FUNCTION F_GetROI : HRESULT
VAR_INPUT
	sFileName 			: 	REFERENCE TO STRING;
	stRoi				:	REFERENCE TO TcVnRectangle_UDINT;
	fThreshold			:	REFERENCE TO LREAL;
	bInvertImage		: 	REFERENCE TO BOOL;
	sPattern			:	REFERENCE TO STRING;
END_VAR
VAR
END_VAR

IF sFileName = 'OCR_01.png' THEN
	stRoi.nX := 86;
	stRoi.nY := 34;
	stRoi.nWidth := 263;
	stRoi.nHeight := 102;
	fThreshold := 150;
	bInvertImage := TRUE;
	sPattern := 'dd#dd#dd';
ELSIF sFileName = 'OCR_02.png' THEN
	stRoi.nX := 69;
	stRoi.nY := 40;
	stRoi.nWidth := 237;
	stRoi.nHeight := 80;
	fThreshold := 150;
	bInvertImage := TRUE;
	sPattern := 'dd#dd#dddd';
ELSIF sFileName = 'OCR_03.png' THEN
	stRoi.nX := 30;
	stRoi.nY := 40;
	stRoi.nWidth := 460;
	stRoi.nHeight := 110;
	fThreshold := 120;
	bInvertImage := TRUE;
	sPattern := 'udddudd###d';
ELSIF sFileName = 'OCR_04.png' THEN
	stRoi.nX := 131;
	stRoi.nY := 25;
	stRoi.nWidth := 243;
	stRoi.nHeight := 83;
	fThreshold := 75;
	bInvertImage := TRUE;
	sPattern := 'dd#dd#dddd';
ELSIF sFileName = 'OCR_05.png' THEN
	stRoi.nX := 129;
	stRoi.nY := 78;
	stRoi.nWidth := 257;
	stRoi.nHeight := 115;
	fThreshold := 150;
	bInvertImage := TRUE;
	sPattern := 'dd#dd#dd';
ELSIF sFileName = 'OCR_06.png' THEN
	stRoi.nX := 71;
	stRoi.nY := 50;
	stRoi.nWidth := 293;
	stRoi.nHeight := 101;
	fThreshold := 75;
	bInvertImage := TRUE;
	sPattern := 'dd#dd#dddd';
ELSIF sFileName = 'OCR_07.png' THEN
	stRoi.nX := 50;
	stRoi.nY := 120;
	stRoi.nWidth := 470;
	stRoi.nHeight := 110;
	fThreshold := 140;
	bInvertImage := FALSE;
	sPattern := 'udddudd###';
ELSIF sFileName = 'OCR_08.png' THEN
	stRoi.nX := 100;
	stRoi.nY := 83;
	stRoi.nWidth := 276;
	stRoi.nHeight := 108;
	fThreshold := 165;
	bInvertImage := TRUE;
	sPattern := 'dd#dd#dd';
ELSIF sFileName = 'OCR_09.png' THEN
	stRoi.nX := 90;
	stRoi.nY := 103;
	stRoi.nWidth := 284;
	stRoi.nHeight := 82; 
	fThreshold := 178;
	bInvertImage := TRUE;
	sPattern := 'dd#dd#dddd';
ELSIF sFileName = 'OCR_10.png' THEN
	stRoi.nX := 207;
	stRoi.nY := 4;
	stRoi.nWidth := 283;
	stRoi.nHeight := 104;
	fThreshold := 130;
	bInvertImage := TRUE;
	sPattern := 'dd#dd#dddd';
ELSIF sFileName = 'OCR_11.png' THEN
	stRoi.nX := 175;
	stRoi.nY := 245;
	stRoi.nWidth := 660;
	stRoi.nHeight := 115;
	fThreshold := 160;
	bInvertImage := TRUE;
	sPattern := 'uu#dddddddd';	
ELSIF sFileName = 'OCR_12.png' THEN 
	stRoi.nX := 74;
	stRoi.nY := 198;
	stRoi.nWidth := 248;
	stRoi.nHeight := 95;
	fThreshold := 130;
	bInvertImage := FALSE;
	sPattern := 'dd#dddd';
ELSIF sFileName = 'OCR_13.png' THEN
	stRoi.nX := 404;
	stRoi.nY := 2;
	stRoi.nWidth := 392;
	stRoi.nHeight := 159;
	fThreshold := 130;
	bInvertImage := FALSE;
	sPattern := 'dd#dd#dd';
ELSIF sFileName = 'OCR_14.png' THEN
	stRoi.nX := 260;
	stRoi.nY := 105;
	stRoi.nWidth := 340;
	stRoi.nHeight := 102;
	fThreshold := 160;
	bInvertImage := FALSE;
	sPattern := 'dd#dd#dddd';
ELSIF sFileName = 'OCR_15.png' THEN
	stRoi.nX := 250;
	stRoi.nY := 5;
	stRoi.nWidth := 560;
	stRoi.nHeight := 125;
	fThreshold := 160;
	bInvertImage := TRUE;
	sPattern := 'uddddd#dd#dd';
ELSIF sFileName = 'OCR_16.png' THEN
	stRoi.nX := 200;
	stRoi.nY := 0;
	stRoi.nWidth := 285;
	stRoi.nHeight := 70;
	fThreshold := 130;
	bInvertImage := FALSE;
	sPattern := 'dd#dd#dddd';
ELSIF sFileName = 'OCR_17.png' THEN
	stRoi.nX := 247;
	stRoi.nY := 83;
	stRoi.nWidth := 213;
	stRoi.nHeight := 94;
	fThreshold := 155;
	bInvertImage := FALSE;
	sPattern := 'dd#dddd';
ELSIF sFileName = 'OCR_18.png' THEN
	stRoi.nX := 25;
	stRoi.nY := 187;
	stRoi.nWidth := 330;
	stRoi.nHeight := 109;
	fThreshold := 100;
	bInvertImage := FALSE;
	sPattern := 'dd#dddd';
ELSIF sFileName = 'OCR_19.png' THEN
	stRoi.nX := 365;
	stRoi.nY := 70;
	stRoi.nWidth := 300;
	stRoi.nHeight := 95;
	fThreshold := 80;
	bInvertImage := TRUE;
	sPattern := 'uduuuud';
END_IF

END_FUNCTION
